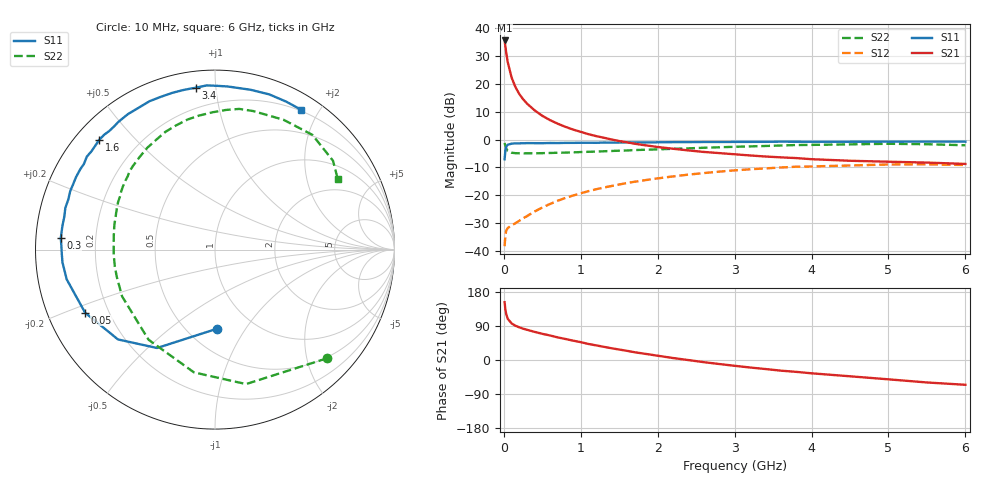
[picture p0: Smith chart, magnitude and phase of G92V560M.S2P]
! SIEMENS Small Signal Semiconductors
! BFG235
! Si NPN RF Bipolar Junction Transistor in SOT223
! VCE = 2.5 V  IC = 60 mA
! Common Emitter S-Parameters:  July  1994
# GHz  S  MA  R  50
!  f  S11  S21  S12  S22
! GHz  MAG  ANG  MAG  ANG  MAG  ANG  MAG  ANG
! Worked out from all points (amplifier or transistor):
!   40 points, 10 MHz to 6 GHz, reference 50 ohm
!   highest |S21| = 35.6 dB at 10 MHz (marker M1)
!   |S21| within 3 dB of that: start of sweep to 24.29 MHz
!   unconditionally stable (mu >= 1): 480.6 MHz to 1.498 GHz
!   at 200 MHz: K = 0.71, MSG = 22.8 dB, |S12| = -29.2 dB
!   at 1.5 GHz: K = 1.00, MSG = 7.8 dB, |S12| = -16.2 dB
!   at 6 GHz: K = 0.94, MSG = 0.2 dB, |S12| = -9.2 dB
!   S11 on the Smith chart (normalised r, x): 10 MHz: 0.69, -0.75; 50 MHz: 0.11, -0.23; 300 MHz: 0.07, +0.04; 1.6 GHz: 0.07, +0.40; 3.4 GHz: 0.09, +0.88; 6 GHz: 0.18, +1.77
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0.01  0.4412 -88.6  60.37 152.5  0.0121 64.7  0.8693 -44.2
0.02  0.6363 -120.5  47.4 133.6  0.0191 48.3  0.7689 -77.0
0.03  0.7367 -137.2  37.24 121.7  0.0227 39.0  0.6941 -99.7
0.05  0.8045 -154.1  24.82 109.0  0.0256 30.2  0.6239 -126.4
0.1  0.8429 -168.7  13.11 96.7  0.0287 30.4  0.5796 -153.2
0.15  0.8529 -175.2  8.809 90.4  0.0312 34.6  0.568 -164.2
0.2  0.8539 -178.5  6.592 86.3  0.0346 38.9  0.5661 -170.3
0.25  0.8567 178.2  5.313 82.7  0.0383 42.7  0.5644 -174.6
0.3  0.8617 175.8  4.441 79.8  0.0419 45.5  0.5648 -178.1
0.4  0.8603 171.2  3.347 74.2  0.0508 49.7  0.5653 176.8
0.5  0.8594 167.6  2.669 69.1  0.06 51.9  0.5687 172.7
0.6  0.8655 164.5  2.233 64.7  0.0694 52.8  0.573 169.0
0.7  0.8637 161.0  1.926 59.7  0.0792 53.2  0.5782 165.6
0.8  0.87 158.0  1.691 55.5  0.0891 52.5  0.5815 162.5
1.1  0.8741 149.0  1.247 42.3  0.1179 49.0  0.6017 153.7
1.6  0.8889 136.5  0.891 24.2  0.1648 40.0  0.6355 139.9
2.2  0.8974 122.7  0.682 5.2  0.2172 27.3  0.6813 123.6
3.2  0.9067 101.0  0.517 -19.8  0.2913 4.2  0.7519 96.8
3.4  0.9083 96.8  0.495 -23.8  0.3029 -0.6  0.7653 91.0
4.5  0.9124 77.4  0.415 -43.0  0.3414 -25.7  0.818 62.1
5.5  0.9149 64.3  0.385 -59.3  0.3582 -47.5  0.823 37.0
6  0.9149 58.5  0.364 -65.4  0.3479 -55.7  0.7885 29.7
